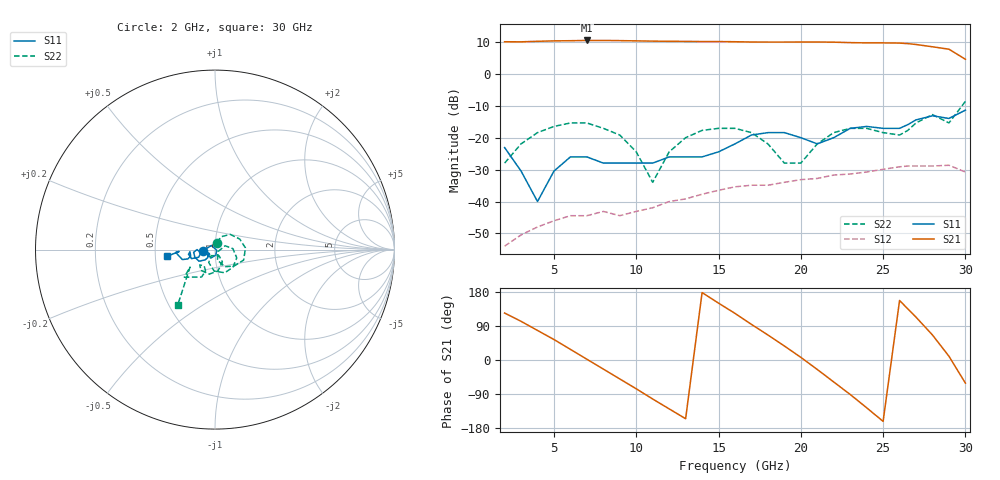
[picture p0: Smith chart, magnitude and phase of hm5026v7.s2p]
! HMMC-5021, HMMC-5022, HMMC-5026
! S-PARAMETERS at  Vdd=7V; Idd=150mA.  LAST UPDATED 02-03-97
# GHZ  S  MA  R  50
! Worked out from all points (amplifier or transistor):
!   30 points, 2 GHz to 30 GHz, reference 50 ohm
!   highest |S21| = 10.4 dB at 7 GHz (marker M1)
!   |S21| within 3 dB of that: start of sweep to 29.08 GHz
!   unconditionally stable (mu >= 1): start of sweep to end of sweep
!   at 7 GHz: K = 24.26, MAG = 10.6 dB, |S12| = -44.4 dB
!   at 17 GHz: K = 8.62, MAG = 10.1 dB, |S12| = -34.9 dB
!   at 30 GHz: K = 8.24, MAG = 5.5 dB, |S12| = -30.8 dB
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2  0.07 -174.0  3.18 124.0  0.002 167.0  0.04 77.0
4  0.01 -20.0  3.23 78.0  0.004 95.0  0.12 45.0
5  0.03 -80.0  3.28 54.0  0.005 67.0  0.15 23.0
7  0.05 -137.0  3.33 2.0  0.006 1.0  0.17 -20.0
8  0.04 -153.0  3.33 -24.0  0.007 -28.0  0.14 -41.0
10  0.04 -141.0  3.28 -76.0  0.007 -54.0  0.06 -77.0
11  0.04 -138.0  3.25 -103.0  0.008 -75.0  0.02 -33.0
12  0.05 -142.0  3.23 -129.0  0.01 -97.0  0.06 21.0
14  0.05 -143.0  3.2 178.0  0.013 -146.0  0.13 -21.0
16  0.08 -134.0  3.18 123.0  0.017 161.0  0.14 -67.0
18  0.12 -159.0  3.14 66.0  0.018 105.0  0.08 -116.0
20  0.1 -180.0  3.15 7.0  0.022 51.0  0.04 -57.0
21  0.08 -168.0  3.15 -25.0  0.023 23.0  0.08 -59.0
22  0.1 -155.0  3.13 -58.0  0.026 -8.0  0.12 -82.0
23  0.14 -159.0  3.08 -91.0  0.027 -40.0  0.14 -103.0
24  0.15 -170.0  3.05 -126.0  0.029 -72.0  0.14 -124.0
25  0.14 -175.0  3.05 -162.0  0.032 -106.0  0.12 -135.0
26  0.14 -165.0  3.03 157.0  0.035 -146.0  0.11 -123.0
27  0.19 -163.0  2.88 113.0  0.036 172.0  0.17 -116.0
28  0.22 -176.0  2.65 66.0  0.036 126.0  0.23 -138.0
29  0.2 -177.0  2.43 10.0  0.037 73.0  0.17 -145.0
30  0.27 -172.0  1.69 -61.0  0.029 5.0  0.37 -124.0
